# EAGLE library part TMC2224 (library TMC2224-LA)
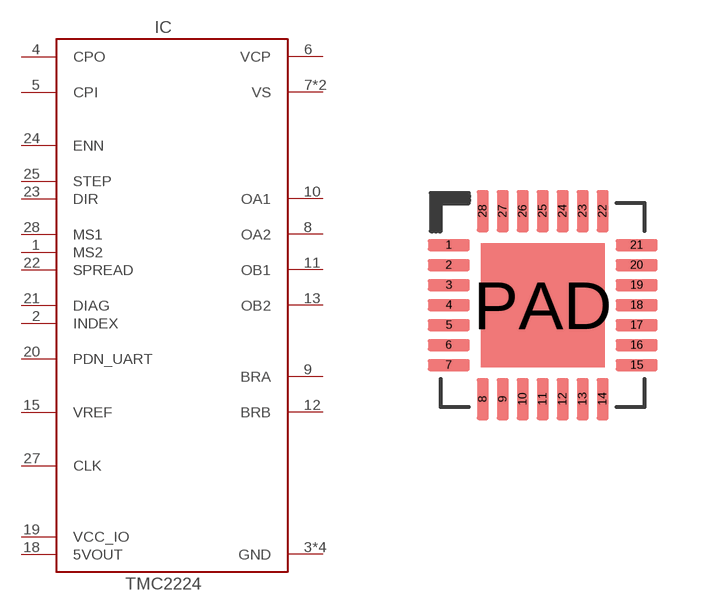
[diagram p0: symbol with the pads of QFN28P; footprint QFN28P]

Designator prefix IC

## TMC2224-LA  [QFN28P]
1  MS2
2  INDEX
3  GND
4  CPO
5  CPI
6  VCP
7  VS
8  OA2
9  BRA
10  OA1
11  OB1
12  BRB
13  OB2
14  VS
15  VREF
16  GND
17  GND
18  5VOUT
19  VCC_IO
20  PDN_UART
21  DIAG
22  SPREAD
23  DIR
24  ENN
25  STEP
27  CLK
28  MS1
PAD  GND

## Footprint QFN28P (pad centres in mm)
smd 1.05 x 0.3: 1 -2.35,1.5; 2 -2.35,1; 3 -2.35,0.5; 4 -2.35,0; 5 -2.35,-0.5; 6 -2.35,-1; 7 -2.35,-1.5; 15 2.35,-1.5; 16 2.35,-1; 17 2.35,-0.5; 18 2.35,0; 19 2.35,0.5; 20 2.35,1; 21 2.35,1.5
smd 0.3 x 1.05: 8 -1.5,-2.35; 9 -1,-2.35; 10 -0.5,-2.35; 11 0,-2.35; 12 0.5,-2.35; 13 1,-2.35; 14 1.5,-2.35; 22 1.5,2.35; 23 1,2.35; 24 0.5,2.35; 25 0,2.35; 26 -0.5,2.35; 27 -1,2.35; 28 -1.5,2.35
smd 3.1 x 3.1: PAD 0,0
